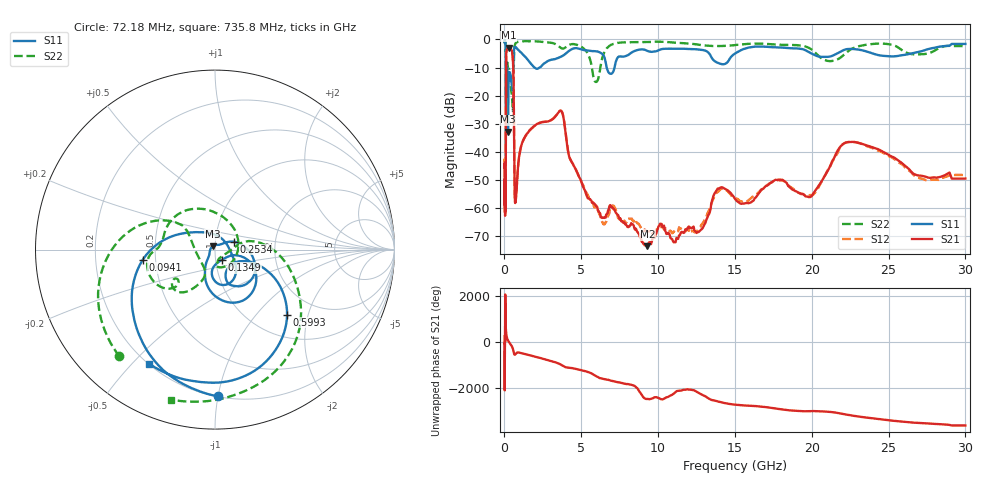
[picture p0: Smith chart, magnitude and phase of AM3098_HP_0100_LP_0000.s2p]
! Date/Time: Thu, Feb 28, 2019 8:34 AM
! Network Analyzer: Agilent Technologies E8364B Rev: A.07.50.67
! Sweep from 0.010 to 30.000 GHz, 1601 Points, Sweep Type: LOG
! Power Supply: 5.022 V, 0.002 A
# Hz S DB R 50
!freq MagS11 AngS11 MagS21 AngS21 MagS12 AngS12 MagS22 AngS22
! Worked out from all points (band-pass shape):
!   1601 points, 10 MHz to 30 GHz, reference 50 ohm
!   highest |S21| = -2.95 dB at 266.5 MHz (marker M1); lowest = -73.8 dB at 9.302 GHz (marker M2)
!   |S21| within 3 dB of the highest: 111.2 MHz to 533.7 MHz (422.6 MHz wide, 131 % of centre)
!   lowest |S11| = -32.9 dB at 230.5 MHz (marker M3), VSWR 1.05, Z = 48.7 + j1.8 ohm
!   |S11| at or under -10 dB: 176.7 MHz to 562.3 MHz (385.6 MHz wide, 104 % of centre); 1.956 GHz to 2.281 GHz (325 MHz wide, 15.3 % of centre); 6.652 GHz to 7.164 GHz (511.2 MHz wide, 7.4 % of centre)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
!   |S22| runs from -25.5 to -0.5 dB; largest |S21 - S12| = 0.011
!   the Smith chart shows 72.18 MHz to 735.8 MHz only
!   S11 on the Smith chart (normalised r, x): 72.18 MHz: 0.20, -1.00; 94.1 MHz: 0.42, -0.06; 134.9 MHz: 1.07, -0.12; 253.4 MHz: 1.23, +0.11; 599.3 MHz: 1.45, -1.48; 735.8 MHz: 0.20, -0.56
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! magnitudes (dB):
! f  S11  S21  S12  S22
! 10 MHz  -0.3  -45.7  -43.7  -0.5
! 38.04 MHz  -0.5  -59.7  -59.9  -0.8
! 72.18 MHz  -1.7  -53.1  -52.8  -2.0
! 94.1 MHz  -7.8  -20.8  -20.9  -9.4
! 134.9 MHz  -23.2  -3.9  -3.9  -11.5
! 144.7 MHz  -16.0  -3.6  -3.6  -10.8
! 187.7 MHz  -11.3  -3.4  -3.4  -8.3
! 230.5 MHz  -32.9  -3.0  -3.0  -10.1
! 253.4 MHz  -18.7  -3.0  -2.9  -10.5
! 266.5 MHz  -15.6  -2.9  -2.9  -10.6
! 550.5 MHz  -12.0  -7.2  -7.2  -25.3
! 599.3 MHz  -5.3  -18.4  -18.4  -10.0
! 665.8 MHz  -2.6  -54.9  -54.8  -2.3
! 735.8 MHz  -2.7  -57.5  -56.8  -1.2
! 2.084 GHz  -10.4  -30.3  -30.3  -0.7
! 3.686 GHz  -6.1  -25.5  -25.4  -3.1
! 5.959 GHz  -4.2  -59.3  -59.9  -15.2
! 7.926 GHz  -5.9  -66.1  -65.2  -1.0
! 9.302 GHz  -4.1  -73.8  -68.4  -0.9
! 19.7 GHz  -4.2  -56.0  -55.8  -2.7
! 22.67 GHz  -3.4  -36.5  -36.5  -3.2
! 30 GHz  -1.6  -49.6  -48.3  -2.3
